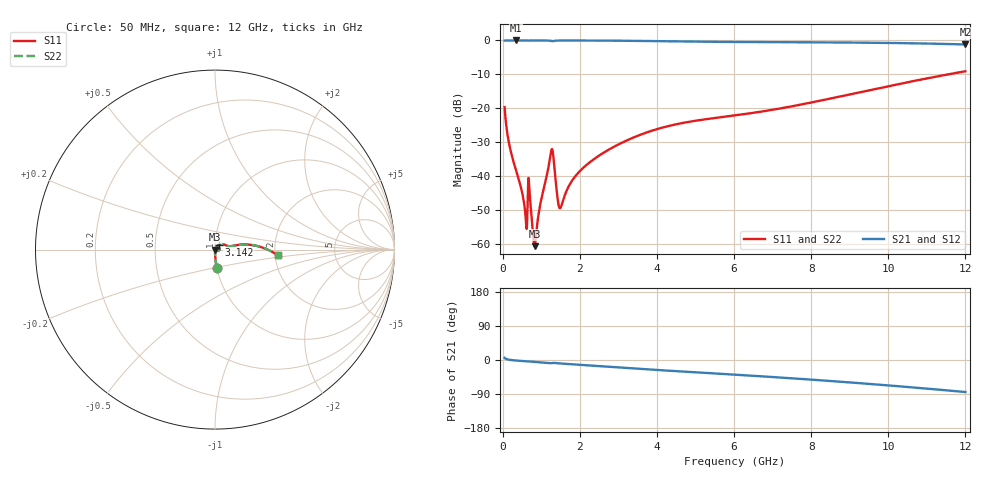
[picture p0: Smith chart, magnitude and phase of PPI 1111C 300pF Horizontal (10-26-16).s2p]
# MHz S MA R 50
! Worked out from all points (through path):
!   1601 points, 50 MHz to 12 GHz, reference 50 ohm
!   highest |S21| = -0.01 dB at 341.3 MHz (marker M1); lowest = -1.2 dB at 12 GHz (marker M2)
!   group delay of S21, straight-line fit = 19.1 ps
!   lowest |S11| = -60.5 dB at 826.8 MHz (marker M3), VSWR 1.00, Z = 50.1 - j0.00587 ohm
!   |S11| at or under -10 dB: start of sweep to 11.54 GHz
!   |S22| runs from -60.5 to -9.1 dB; largest |S21 - S12| = 0
!   S11 on the Smith chart (normalised r, x): 50 MHz: 1.00, -0.21; 3.142 GHz: 1.04, +0.05; 12 GHz: 2.07, -0.15
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50  0.1046 -84.2  0.9943 5.7  0.9943 5.7  0.1046 -84.2
176.9688  0.02836 -88.7  0.9992 0.6  0.9992 0.6  0.02836 -88.7
341.2812  0.01257 -89.1  0.9994 -1.3  0.9994 -1.3  0.01257 -89.1
490.6562  0.006269 -87.1  0.9993 -2.6  0.9993 -2.6  0.006269 -87.1
580.2812  0.003107 -77.9  0.9991 -3.3  0.9991 -3.3  0.003107 -77.9
707.25  0.004857 -69.9  0.998 -4.0  0.998 -4.0  0.004857 -69.9
781.9375  0.001564 -55.4  0.999 -4.7  0.999 -4.7  0.001564 -55.4
826.75  0.0009431 -3.6  0.999 -5.0  0.999 -5.0  0.0009431 -3.6
864.0938  0.001351 39.9  0.999 -5.3  0.999 -5.3  0.001351 39.9
998.5312  0.004522 68.1  0.9987 -6.3  0.9987 -6.3  0.004522 68.1
1259.938  0.02395 29.9  0.981 -8.5  0.981 -8.5  0.02395 29.9
1312.219  0.02008 -18.8  0.9802 -7.7  0.9802 -7.7  0.02008 -18.8
1424.25  0.004715 -24.5  0.9954 -8.5  0.9954 -8.5  0.004715 -24.5
1491.469  0.003418 16.8  0.9968 -9.1  0.9968 -9.1  0.003418 16.8
1752.875  0.007871 62.8  0.9977 -11.0  0.9977 -11.0  0.007871 62.8
2044.156  0.01266 65.0  0.9972 -13.0  0.9972 -13.0  0.01266 65.0
3142.062  0.03231 52.0  0.9896 -20.6  0.9896 -20.6  0.03231 52.0
4038.312  0.05031 36.1  0.9756 -26.5  0.9756 -26.5  0.05031 36.1
6025  0.07907 13.6  0.9494 -38.7  0.9494 -38.7  0.07907 13.6
8019.156  0.1228 11.7  0.9389 -51.9  0.9389 -51.9  0.1228 11.7
10013.31  0.213 6.7  0.919 -67.2  0.919 -67.2  0.213 6.7
12000  0.3522 -5.2  0.8721 -84.5  0.8721 -84.5  0.3522 -5.2
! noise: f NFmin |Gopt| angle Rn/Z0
50  0.0003431  0.8556  0.3758  0.0005075
1372  0.009996  0.8639  8.278  0.01568
2701  0.01197  0.7881  16.16  0.0114
4031  0.0292  0.8675  23.91  0.04535
5360  0.04589  0.8897  31.43  0.08392
6682  0.0552  0.8896  38.62  0.09693
8012  0.06135  0.8858  45.52  0.09926
9341  0.06696  0.8835  52.07  0.1007
1.067e+04  0.0729  0.8834  58.26  0.1036
1.2e+04  0.0795  0.8856  64.1  0.1086
